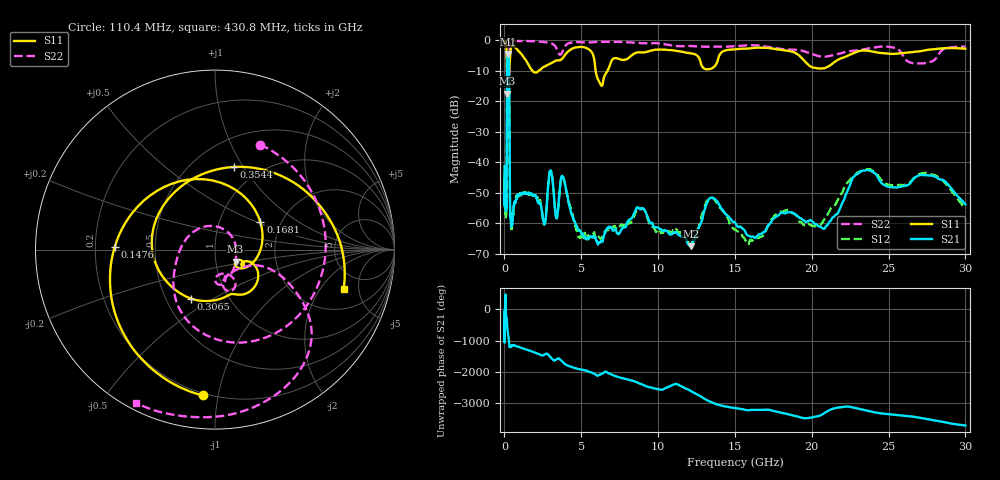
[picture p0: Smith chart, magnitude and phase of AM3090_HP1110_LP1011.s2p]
! Date/Time: Thu, Feb 28, 2019 2:09 PM
! Network Analyzer: Agilent Technologies E8364B Rev: A.07.50.67
! Sweep from 0.010 to 30.000 GHz, 1601 Points, Sweep Type: LOG
! Power Supply: 5.022 V, 0.002 A
# Hz S DB R 50
!freq MagS11 AngS11 MagS21 AngS21 MagS12 AngS12 MagS22 AngS22
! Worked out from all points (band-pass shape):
!   1601 points, 10 MHz to 30 GHz, reference 50 ohm
!   highest |S21| = -4.58 dB at 225.9 MHz (marker M1); lowest = -67.6 dB at 12.13 GHz (marker M2)
!   |S21| within 3 dB of the highest: 176.4 MHz to 289.4 MHz (113.1 MHz wide, 48.6 % of centre)
!   lowest |S11| = -17.5 dB at 193.4 MHz (marker M3), VSWR 1.31, Z = 62.3 - j8.48 ohm
!   |S11| at or under -10 dB: 166.2 MHz to 313 MHz (146.8 MHz wide, 61.3 % of centre); 1.812 GHz to 2.239 GHz (427.3 MHz wide, 21.1 % of centre); 5.93 GHz to 6.72 GHz (789.8 MHz wide, 12.5 % of centre)
!   |S22| runs from -18.6 to -0.1 dB; largest |S21 - S12| = 0.011
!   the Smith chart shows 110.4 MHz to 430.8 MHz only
!   S11 on the Smith chart (normalised r, x): 110.4 MHz: 0.19, -0.90; 147.6 MHz: 0.28, +0.01; 168.1 MHz: 1.57, +0.53; 306.5 MHz: 0.67, -0.40; 354.4 MHz: 0.77, +0.91; 430.8 MHz: 3.37, -3.42
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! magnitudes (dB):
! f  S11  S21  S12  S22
! 10 MHz  -0.3  -41.3  -46.5  -0.6
! 38.04 MHz  -0.3  -50.4  -50.7  -1.4
! 110.4 MHz  -1.8  -53.0  -53.4  -3.9
! 144.7 MHz  -4.5  -47.1  -47.8  -4.9
! 147.6 MHz  -5.1  -43.5  -44.2  -5.3
! 168.1 MHz  -10.6  -11.7  -11.7  -18.4
! 193.4 MHz  -17.5  -5.3  -5.2  -15.6
! 225.9 MHz  -15.5  -4.6  -4.5  -16.5
! 306.5 MHz  -10.4  -13.7  -13.6  -7.7
! 354.4 MHz  -6.5  -52.6  -52.1  -0.8
! 430.8 MHz  -2.5  -61.0  -60.2  -0.3
! 550.5 MHz  -2.0  -57.5  -58.3  -0.3
! 2.084 GHz  -10.7  -51.9  -51.4  -0.5
! 2.61 GHz  -8.7  -60.4  -60.2  -0.7
! 3.002 GHz  -7.7  -42.7  -42.8  -1.1
! 4.952 GHz  -2.3  -62.6  -64.3  -0.7
! 7.926 GHz  -6.3  -60.9  -60.3  -0.7
! 12.13 GHz  -4.4  -67.6  -66.4  -2.0
! 13.54 GHz  -9.2  -51.7  -51.9  -2.2
! 20.82 GHz  -9.2  -61.9  -58.7  -5.4
! 23.36 GHz  -3.4  -42.8  -42.5  -3.1
! 30 GHz  -2.8  -53.8  -55.1  -2.2
